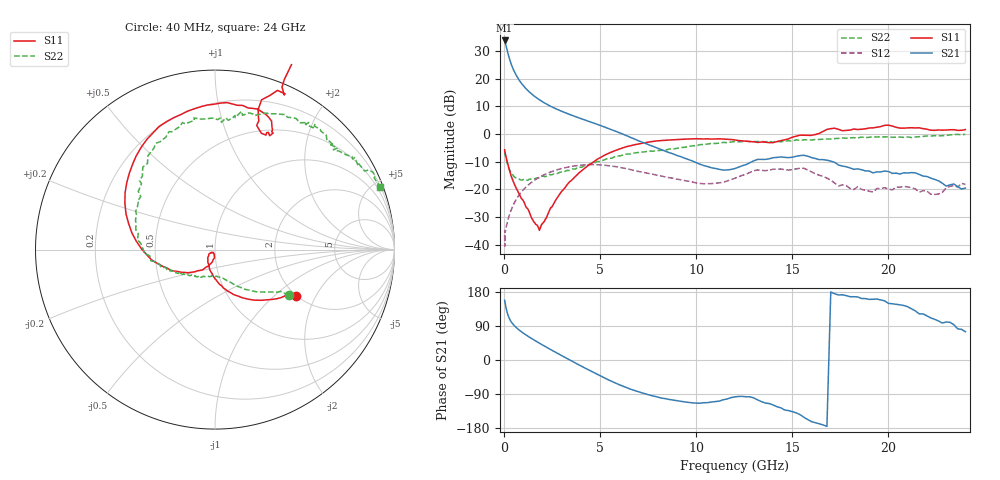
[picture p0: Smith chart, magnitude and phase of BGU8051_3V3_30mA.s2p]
! BGU8051_3V3_30mA
! Date/time Tue Jun 16 10:58:09 2015
! VAR V_out= 3.3000
! VAR I_out= 29.9850
! VAR V_in= 3.8490
! VAR I_in= 0.4079
# MHz S MA R 50
!  Freq-MHz  S11-mag  S11-arg  S21-mag  S21-arg  S12-mag  S12-arg  S22-mag  S22-arg
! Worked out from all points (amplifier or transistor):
!   187 points, 40 MHz to 24 GHz, reference 50 ohm
!   highest |S21| = 33.7 dB at 40 MHz (marker M1)
!   |S21| within 3 dB of that: start of sweep to 153.4 MHz
!   unconditionally stable (mu >= 1): 636.7 MHz to 13.31 GHz; 13.45 GHz to 14.03 GHz
!   at 750 MHz: K = 1.01, MAG = 20.6 dB, |S12| = -22.4 dB
!   at 5.4 GHz: K = 1.21, MAG = 4.0 dB, |S12| = -11.4 dB
!   at 24 GHz: K = 0.28, MSG = -0.7 dB, |S12| = -18.2 dB
!   lowest NFmin = 0.28 dB at 400 MHz
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40  0.5189 -30.0  48.62 157.5  0.01505 31.6  0.4836 -31.6
60  0.472 -32.7  46.37 152.1  0.01829 55.9  0.4347 -32.4
80  0.441 -38.3  43.27 146.6  0.01742 38.8  0.4015 -36.1
120  0.3814 -47.8  38.34 136.3  0.02016 43.5  0.3496 -42.5
140  0.3548 -52.5  36.03 131.8  0.02232 45.5  0.3299 -45.4
180  0.3089 -60.4  31.58 124.1  0.02571 48.8  0.2937 -50.1
240  0.2551 -70.1  26.3 115.0  0.03045 53.0  0.2537 -56.0
300  0.2178 -77.9  22.3 108.1  0.03535 55.1  0.2257 -60.5
360  0.1847 -84.7  19.22 102.7  0.04071 57.1  0.2043 -64.0
440  0.1529 -92.3  16.17 96.8  0.04781 58.2  0.1864 -68.8
550  0.1238 -101.4  13.25 90.2  0.05779 58.8  0.1679 -73.6
750  0.08983 -113.3  9.914 81.0  0.07556 57.6  0.1552 -81.2
950  0.06662 -126.8  7.913 73.2  0.09321 55.0  0.1478 -87.8
1600  0.02528 -140.9  4.774 51.8  0.1473 43.0  0.1558 -107.5
2600  0.05567 -99.8  2.963 22.9  0.2162 21.5  0.1911 -129.5
4100  0.2234 -145.4  1.848 -18.1  0.2756 -12.2  0.2555 -151.8
6200  0.5648 152.8  0.9901 -69.3  0.244 -54.9  0.4156 175.1
8200  0.7629 110.5  0.5211 -100.5  0.1741 -75.9  0.5075 148.2
12200  0.7623 65.4  0.2516 -96.1  0.1691 -70.6  0.7204 103.3
16200  0.9794 67.6  0.3612 -165.5  0.1921 -150.0  0.7968 71.3
20200  1.391 32.7  0.1946 148.5  0.09826 -148.8  0.8697 44.2
24000  1.2 20.1  0.1059 74.8  0.1234 -164.1  0.9852 20.7
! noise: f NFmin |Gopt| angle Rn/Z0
400  0.281  0.1956  27.47  0.0531
550  0.2966  0.1611  35.56  0.0532
950  0.3476  0.09993  71.27  0.0526
1250  0.395  0.09283  108.4  0.0515
1600  0.4603  0.115  140.3  0.0501
1900  0.5247  0.1411  156.8  0.0492
2250  0.6097  0.1703  170.1  0.049
2600  0.7053  0.1964  180.5  0.0503
3300  0.9286  0.2434  197.9  0.0597
4000  1.194  0.292  212.2  0.0819
